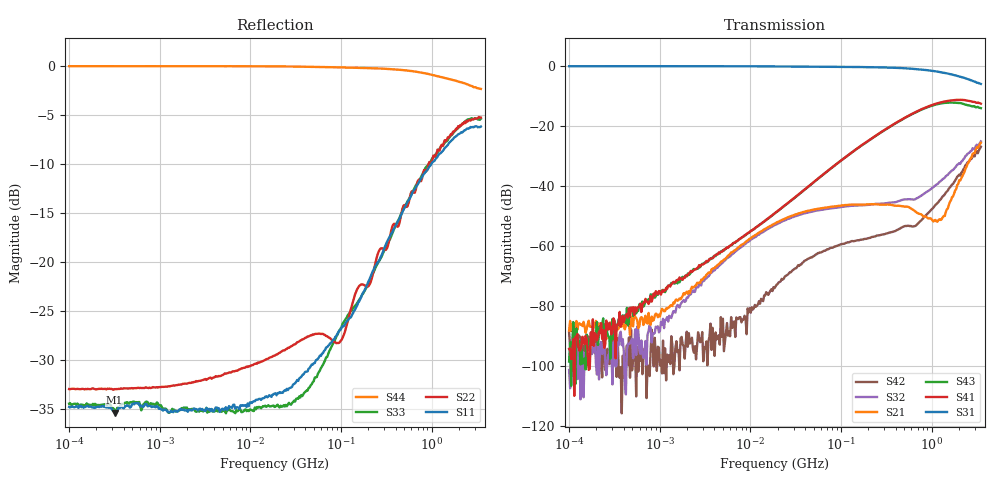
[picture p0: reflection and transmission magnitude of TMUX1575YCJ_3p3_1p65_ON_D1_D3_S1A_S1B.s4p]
!Keysight Technologies,E5080A,MY55200740,A.12.60.03
!Date: Tuesday, July 21, 2020 15:01:57
!Correction: S11(Full 4 Port(1,2,3,4))
!S12(Full 4 Port(1,2,3,4))
!S13(Full 4 Port(1,2,3,4))
!S14(Full 4 Port(1,2,3,4))
!S21(Full 4 Port(1,2,3,4))
!S22(Full 4 Port(1,2,3,4))
!S23(Full 4 Port(1,2,3,4))
!S24(Full 4 Port(1,2,3,4))
!S31(Full 4 Port(1,2,3,4))
!S32(Full 4 Port(1,2,3,4))
!S33(Full 4 Port(1,2,3,4))
!S34(Full 4 Port(1,2,3,4))
!S41(Full 4 Port(1,2,3,4))
!S42(Full 4 Port(1,2,3,4))
!S43(Full 4 Port(1,2,3,4))
!S44(Full 4 Port(1,2,3,4))
!S4P File: Measurements: <S11,S12,S13,S14>,
!<S21,S22,S23,S24>,
!<S31,S32,S33,S34>,
!<S41,S42,S43,S44>:Log Frequency Sweep
# Hz S  dB  R 50
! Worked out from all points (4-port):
!   400 points, 100 kHz to 3.5 GHz, reference 50 ohm
!   strongest paths, dB at 100 kHz, 1.377 MHz, 18.96 MHz, 261 MHz, 3.5 GHz:
!     S31: -0.2, -0.1, -0.2, -0.5, -6.1
!     S41: -94.3, -72.4, -48.9, -22.6, -12.6
!     S43: -98.5, -72.5, -49.0, -22.7, -14.1
!     S21: -88.1, -80.0, -52.4, -46.2, -25.6
!     S32: -101.3, -82.8, -52.9, -45.9, -25.2
!     S42: -88.8, -92.9, -73.5, -56.5, -26.9
!   lowest |S11| = -35.3 dB at 317 kHz (marker M1), VSWR 1.03, Z = 51.7 + j0.368 ohm
!   |S11| at or under -10 dB: start of sweep to 989.4 MHz
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100000  -34.76 8.8  -97.84 -71.1  -0.16 -0.0  -90.78 98.2
        -88.12 -178.6  -32.94 2.9  -86.53 -165.8  -94.78 -101.9
        -0.16 -0.0  -101.26 170.7  -34.42 7.3  -88.74 151.8
        -94.29 89.4  -88.80 -178.8  -98.46 143.6  0.00 -0.0
317029.9  -35.34 12.0  -93.12 96.0  -0.16 -0.1  -83.51 83.5
          -86.37 -178.4  -32.94 3.8  -86.67 -176.7  -97.45 90.5
          -0.16 -0.0  -95.30 130.8  -35.12 8.3  -83.20 82.4
          -84.80 90.7  -96.24 -8.0  -85.05 122.8  0.00 -0.0
1611373  -35.14 -6.1  -80.43 116.5  -0.15 -0.2  -71.44 89.9
         -78.00 156.2  -32.49 2.0  -78.38 163.5  -99.84 125.2
         -0.15 -0.1  -79.93 124.7  -35.16 -8.0  -71.77 91.5
         -71.30 91.9  -94.77 119.2  -71.07 99.3  0.00 -0.1
1.279083e7  -33.93 -38.1  -55.32 79.7  -0.20 -0.9  -52.73 99.2
            -55.27 88.0  -30.20 -23.8  -55.92 87.7  -79.83 109.6
            -0.20 -0.9  -55.90 80.1  -34.79 -39.9  -52.88 99.0
            -52.87 98.8  -79.23 109.1  -52.79 99.3  -0.01 -1.0
9.634388e7  -26.95 -94.1  -46.63 20.6  -0.38 -3.4  -31.90 96.0
            -46.61 21.4  -28.19 -97.6  -47.11 11.7  -59.60 44.5
            -0.37 -3.4  -47.13 10.9  -26.96 -96.5  -31.96 96.8
            -31.94 95.9  -59.62 44.5  -31.96 97.0  -0.12 -6.2
1.163443e9  -9.23 -122.5  -51.94 -64.0  -1.97 -26.8  -12.48 33.0
            -51.89 -64.4  -8.51 -117.4  -39.38 -81.2  -45.71 -50.8
            -1.97 -26.9  -39.37 -81.5  -8.80 -117.9  -12.80 43.6
            -12.47 33.0  -45.70 -50.9  -12.78 43.7  -1.01 -56.5
3.5e9  -6.15 -156.7  -25.66 161.2  -6.09 -50.6  -12.68 -16.6
       -25.62 161.1  -5.24 -142.1  -25.16 -173.8  -27.00 -165.2
       -6.07 -50.8  -25.17 -174.1  -5.36 -144.1  -14.14 36.1
       -12.62 -16.6  -26.94 -165.5  -14.12 36.2  -2.32 -104.1
